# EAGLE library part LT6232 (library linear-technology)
215MHz, Rail-to-Rail Output, 1.1nV/Hz, 3.5mA Op Amp Source: http://cds.linear.com/docs/Datasheet/623012fb.pdf
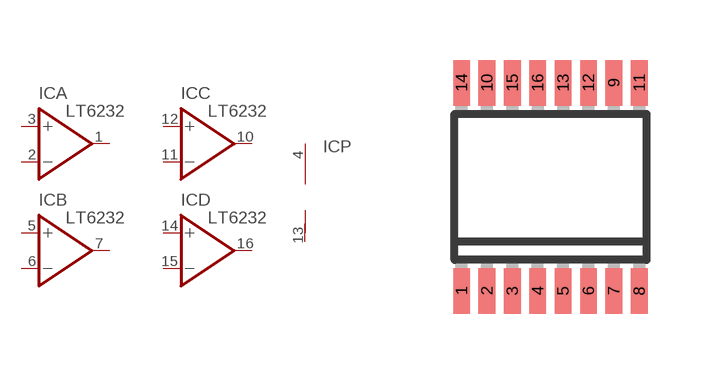
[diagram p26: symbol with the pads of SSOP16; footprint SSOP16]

Designator prefix IC; gates A=OPAMP B=OPAMP C=OPAMP D=OPAMP P=V+-

## LT6232CGN (MPN: LT6232CGN; OC_FARNELL: unknown; OC_NEWARK: 57M9360), LT6232IGN (MPN: LT6232IGN; OC_FARNELL: unknown; OC_NEWARK: 57M9364)  [SSOP16]
1  A:OUT  out
2  A:-IN  in
3  A:+IN  in
4  P:V+  pwr
5  B:+IN  in
6  B:-IN  in
7  B:OUT  out
10  C:OUT  out
11  C:-IN  in
12  C:+IN  in
13  P:V-  pwr
14  D:+IN  in
15  D:-IN  in
16  D:OUT  out

## Footprint SSOP16 (pad centres in mm)
GN Package 16-Lead Plastic SSOP (Narrow .150 Inch) Source: http://cds.linear.com/docs/Datasheet/623012fb.pdf
smd 0.419 x 1.143: 1 -2.223,-2.6; 2 -1.587,-2.6; 3 -0.953,-2.6; 4 -0.318,-2.6; 5 0.318,-2.6; 6 0.953,-2.6; 7 1.587,-2.6; 8 2.223,-2.6; 9 1.587,2.6; 10 -1.587,2.6; 11 2.223,2.6; 12 0.953,2.6; 13 0.318,2.6; 14 -2.223,2.6; 15 -0.953,2.6; 16 -0.318,2.6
